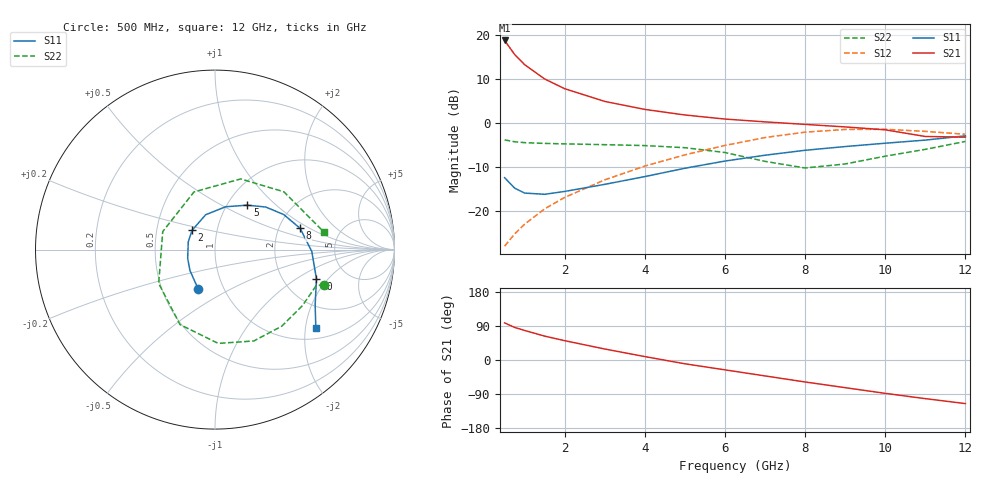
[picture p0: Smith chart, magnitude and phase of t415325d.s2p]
!AT-41532
!S-PARAMETERS at Vce=5V  Ic=10mA.  LAST UPDATED 05-29-98
# ghz s ma r 50
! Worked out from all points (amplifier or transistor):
!   15 points, 500 MHz to 12 GHz, reference 50 ohm
!   highest |S21| = 18.7 dB at 500 MHz (marker M1)
!   |S21| within 3 dB of that: start of sweep to 736 MHz
!   unconditionally stable (mu >= 1): 728.8 MHz to 2.075 GHz
!   at 1 GHz: K = 1.04, MAG = 16.8 dB, |S12| = -23.0 dB
!   at 5 GHz: K = 0.79, MSG = 4.5 dB, |S12| = -7.3 dB
!   at 12 GHz: K = 0.99, MSG = -0.3 dB, |S12| = -2.6 dB
!   S11 on the Smith chart (normalised r, x): 500 MHz: 0.76, -0.35; 2 GHz: 0.76, +0.17; 5 GHz: 1.23, +0.67; 8 GHz: 2.62, +0.82; 10 GHz: 3.04, -1.51; 12 GHz: 1.28, -2.28
0.5  0.239 -113.0  8.601 98.0  0.04 69.0  0.641 -18.0
0.75  0.182 -140.0  5.966 86.0  0.055 70.0  0.611 -19.0
1  0.16 -162.0  4.571 78.0  0.071 71.0  0.597 -20.0
1.5  0.155 164.0  3.144 63.0  0.106 69.0  0.585 -26.0
2  0.167 140.0  2.44 51.0  0.143 66.0  0.578 -33.0
3  0.201 105.0  1.751 29.0  0.226 57.0  0.566 -49.0
4  0.246 76.0  1.421 9.0  0.324 45.0  0.553 -67.0
5  0.306 54.0  1.229 -10.0  0.434 31.0  0.523 -88.0
6  0.369 40.0  1.105 -26.0  0.555 14.0  0.461 -115.0
7  0.43 27.0  1.027 -42.0  0.682 -5.0  0.366 -149.0
8  0.489 14.0  0.961 -58.0  0.785 -26.0  0.308 161.0
9  0.539 -1.0  0.9 -73.0  0.842 -47.0  0.342 110.0
10  0.588 -16.0  0.834 -88.0  0.846 -68.0  0.419 70.0
11  0.638 -29.0  0.701 -102.0  0.801 -88.0  0.501 40.0
12  0.713 -38.0  0.689 -115.0  0.743 -104.0  0.616 9.0
